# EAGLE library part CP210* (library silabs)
Single-Chip USB to UART Bridge Source: www.silabs.com .. CP2101.pdf / cp2102.pdf
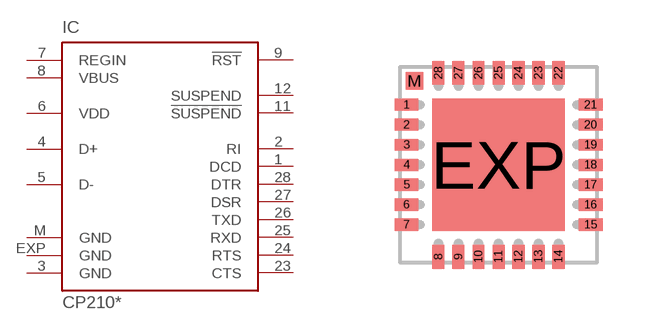
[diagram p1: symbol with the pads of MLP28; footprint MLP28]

Designator prefix IC

## CP2101 (MF: FARNELL; MPN: CP2102-GM; OC_FARNELL: 9282130; OC_NEWARK: 30K5635), CP2102 (MF: FARNELL; MPN: CP2102-GM; OC_FARNELL: 9282130; OC_NEWARK: 30K5635)  [MLP28]
1  DCD  in
2  RI  in
3  GND  pwr
4  D+
5  D-
6  VDD  pwr
7  REGIN  pas
8  VBUS  in
9  !RST
11  !SUSPEND  out
12  SUSPEND  out
23  CTS  in
24  RTS  out
25  RXD  in
26  TXD  out
27  DSR  in
28  DTR  out
EXP  GND  pwr
M  GND  pwr

## Footprint MLP28 (pad centres in mm)
MLP 28 Source: www.silabs.com .. CP2101.pdf
smd 0.6 x 0.3: 1 -2.3,1.5; 2 -2.3,1; 3 -2.3,0.5; 4 -2.3,0; 5 -2.3,-0.5; 6 -2.3,-1; 7 -2.3,-1.5; 15 2.3,-1.5; 16 2.3,-1; 17 2.3,-0.5; 18 2.3,0; 19 2.3,0.5; 20 2.3,1; 21 2.3,1.5
smd 0.3 x 0.6: 8 -1.5,-2.3; 9 -1,-2.3; 10 -0.5,-2.3; 11 0,-2.3; 12 0.5,-2.3; 13 1,-2.3; 14 1.5,-2.3; 22 1.5,2.3; 23 1,2.3; 24 0.5,2.3; 25 0,2.3; 26 -0.5,2.3; 27 -1,2.3; 28 -1.5,2.3
smd 3.3 x 3.3: EXP 0,0
smd 0.435 x 0.435: M -2.103,2.103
